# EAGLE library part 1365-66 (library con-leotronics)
DUAL ROW STRAIGHT HEADER 1364 SERIES. 1.27mm x 1.27mm. Without Fixing Post. SMT Source: http://www.leotronics.co.uk/Conexcon/Data%20Sheets/sec.%20A/1364ing.pdf
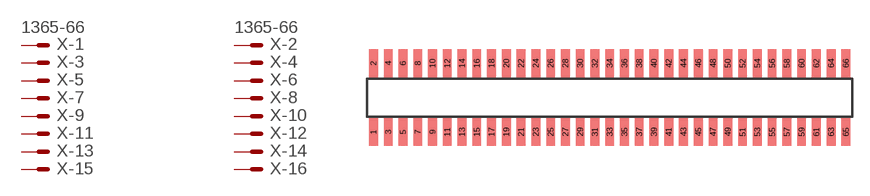
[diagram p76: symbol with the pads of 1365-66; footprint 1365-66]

Designator prefix X; gates -1=MVAL -2=MVAL -3=M -4=M -5=M -6=M -7=M -8=M -9=M -10=M -11=M -12=M -13=M -14=M -15=M -16=M -17=M -18=M -19=M -20=M -21=M -22=M -23=M -24=M -25=M -26=M -27=M -28=M -29=M -30=M -31=M -32=M -33=M -34=M -35=M -36=M -37=M -38=M -39=M -40=M -41=M -42=M -43=M -44=M -45=M -46=M -47=M -48=M -49=M -50=M -51=M -52=M -53=M -54=M -55=M -56=M -57=M -58=M -59=M -60=M -61=M -62=M -63=M -64=M -65=M -66=M

## 1365-66 (OC_FARNELL: unknown; OC_NEWARK: unknown)  [1365-66]
1  -1:S  pas
2  -2:S  pas
3  -3:S  pas
4  -4:S  pas
5  -5:S  pas
6  -6:S  pas
7  -7:S  pas
8  -8:S  pas
9  -9:S  pas
10  -10:S  pas
11  -11:S  pas
12  -12:S  pas
13  -13:S  pas
14  -14:S  pas
15  -15:S  pas
16  -16:S  pas
17  -17:S  pas
18  -18:S  pas
19  -19:S  pas
20  -20:S  pas
21  -21:S  pas
22  -22:S  pas
23  -23:S  pas
24  -24:S  pas
25  -25:S  pas
26  -26:S  pas
27  -27:S  pas
28  -28:S  pas
29  -29:S  pas
30  -30:S  pas
31  -31:S  pas
32  -32:S  pas
33  -33:S  pas
34  -34:S  pas
35  -35:S  pas
36  -36:S  pas
37  -37:S  pas
38  -38:S  pas
39  -39:S  pas
40  -40:S  pas
41  -41:S  pas
42  -42:S  pas
43  -43:S  pas
44  -44:S  pas
45  -45:S  pas
46  -46:S  pas
47  -47:S  pas
48  -48:S  pas
49  -49:S  pas
50  -50:S  pas
51  -51:S  pas
52  -52:S  pas
53  -53:S  pas
54  -54:S  pas
55  -55:S  pas
56  -56:S  pas
57  -57:S  pas
58  -58:S  pas
59  -59:S  pas
60  -60:S  pas
61  -61:S  pas
62  -62:S  pas
63  -63:S  pas
64  -64:S  pas
65  -65:S  pas
66  -66:S  pas

## Footprint 1365-66 (pad centres in mm)
DUAL ROW STRAIGHT HEADER 1364 SERIES. 1.27mm x 1.27mm. Without Fixing Post. SMT Source: http://www.leotronics.co.uk/Conexcon/Data%20Sheets/sec.%20A/1364ing.pdf
smd 0.76 x 2.4: 1 -20.32,-2.95; 2 -20.32,2.95; 3 -19.05,-2.95; 4 -19.05,2.95; 5 -17.78,-2.95; 6 -17.78,2.95; 7 -16.51,-2.95; 8 -16.51,2.95; 9 -15.24,-2.95; 10 -15.24,2.95; 11 -13.97,-2.95; 12 -13.97,2.95; 13 -12.7,-2.95; 14 -12.7,2.95; 15 -11.43,-2.95; 16 -11.43,2.95; 17 -10.16,-2.95; 18 -10.16,2.95; 19 -8.89,-2.95; 20 -8.89,2.95; 21 -7.62,-2.95; 22 -7.62,2.95; 23 -6.35,-2.95; 24 -6.35,2.95; 25 -5.08,-2.95; 26 -5.08,2.95; 27 -3.81,-2.95; 28 -3.81,2.95; 29 -2.54,-2.95; 30 -2.54,2.95; 31 -1.27,-2.95; 32 -1.27,2.95; 33 0,-2.95; 34 0,2.95; 35 1.27,-2.95; 36 1.27,2.95; 37 2.54,-2.95; 38 2.54,2.95; 39 3.81,-2.95; 40 3.81,2.95; 41 5.08,-2.95; 42 5.08,2.95; 43 6.35,-2.95; 44 6.35,2.95; 45 7.62,-2.95; 46 7.62,2.95; 47 8.89,-2.95; 48 8.89,2.95; 49 10.16,-2.95; 50 10.16,2.95; 51 11.43,-2.95; 52 11.43,2.95; 53 12.7,-2.95; 54 12.7,2.95; 55 13.97,-2.95; 56 13.97,2.95; 57 15.24,-2.95; 58 15.24,2.95; 59 16.51,-2.95; 60 16.51,2.95; 61 17.78,-2.95; 62 17.78,2.95; 63 19.05,-2.95; 64 19.05,2.95; 65 20.32,-2.95; 66 20.32,2.95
